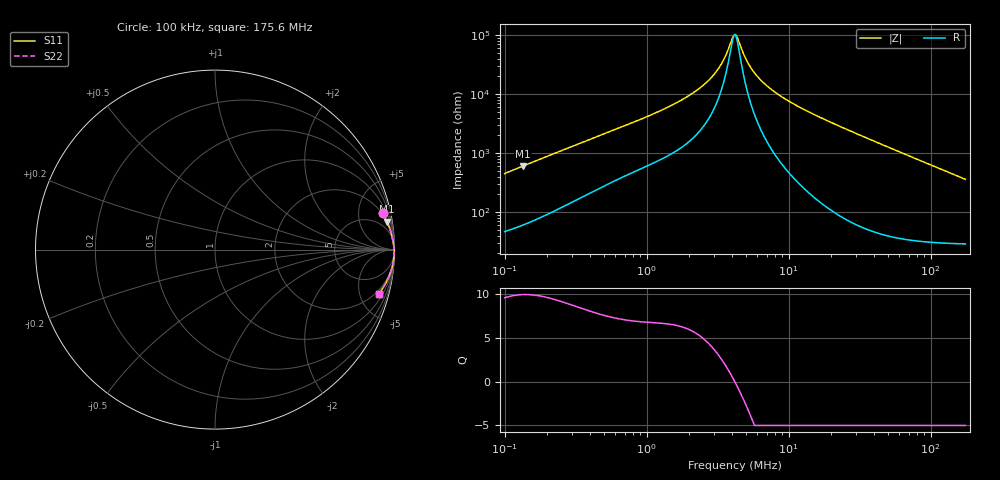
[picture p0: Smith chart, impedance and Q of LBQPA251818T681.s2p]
! LBQPA251818T681  S-PARAMETER MODEL  ( General Type )
! Model Generated by TAIYO YUDEN Corporation (http://www.ty-top.com)
! Version 1.0
! TAIYO YUDEN Control No. 191025NI43SB-FBB
! Copyright(c) 2019 TAIYO YUDEN CO.,LTD. All Rights Reserved.
! Product Description (link to TY-COMPAS)
! https://ds.yuden.co.jp/TYCOMPAS/or/detail?pn=LBQPA251818T681K&u=M
! Products Name : Inductors
! Characteristics :
!  Inductance : 680 uH , SRF(min) : 3.0 MHz , DC Resistance(max) : 36.4 Ohm
!  Rated Current : Saturation :65 mA , Temp Rise : 45 mA (20 degC)
!  Case Size : 2.5 x 1.8 / 0.098 x 0.071 [mm/inch] , Thickness : 1.8 / 0.071 [mm/inch]
!  (Conditions: Temperature = 25 degC , DC Bias Current/Voltage = 0A / 0V)
! External Node Assignments :
!  1  o---GGG---o  2
! GND o---------o GND
! Frequency Range : 0.1MHz  -  175.64884MHz  [ 402 STEP ]
# MHz S RI R 50
! Freq[MHz].  S11 Real  S11 Imag  S21 Real  S21 Imag  S12 Real  S12 Imag  S22 Real  S22 Imag
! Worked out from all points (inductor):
!   401 points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, 100 kHz to 175.6 MHz, reference 50 ohm
!   read as one part in series: L = 710 uH near 103.8 kHz
!   highest Q = 9.95 at 134.8 kHz (marker M1), where L = 710 uH
!   self-resonance near 4.113 MHz
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0.1  0.9342 0.2012  0.0658 -0.2012  0.0658 -0.2012  0.9342 0.2012
0.13483  0.9586 0.1552  0.0414 -0.1552  0.0414 -0.1552  0.9586 0.1552
0.349525  0.988 0.0646  0.012 -0.0646  0.012 -0.0646  0.988 0.0646
1.221676  0.9967 0.0193  0.00326 -0.0193  0.00326 -0.0193  0.9967 0.0193
1.948707  0.9981 0.0107  0.0019 -0.0107  0.0019 -0.0107  0.9981 0.0107
2.676973  0.9986 0.00596  0.00136 -0.00596  0.00136 -0.00596  0.9986 0.00596
2.994426  0.9988 0.00442  0.00123 -0.00442  0.00123 -0.00442  0.9988 0.00442
3.287545  0.9989 0.00316  0.00114 -0.00316  0.00114 -0.00316  0.9989 0.00316
3.609356  0.9989 0.00192  0.00106 -0.00192  0.00106 -0.00192  0.9989 0.00192
4.037378  0.999 0.000448  0.000993 -0.000448  0.000993 -0.000448  0.999 0.000448
4.191048  0.999 -4.2e-05  0.000974 4.2e-05  0.000974 4.2e-05  0.999 -4.2e-05
4.270063  0.999 -0.000287  0.000965 0.000287  0.000965 0.000287  0.999 -0.000287
4.432589  0.9991 -0.000778  0.000948 0.000778  0.000948 0.000778  0.9991 -0.000778
4.866487  0.9991 -0.00202  0.000913 0.00202  0.000913 0.00202  0.9991 -0.00202
5.243992  0.9991 -0.00302  0.000893 0.00302  0.000893 0.00302  0.9991 -0.00302
5.757316  0.9991 -0.0043  0.000877 0.0043  0.000877 0.0043  0.9991 -0.0043
6.440058  0.9991 -0.00589  0.00087 0.00589  0.00087 0.00589  0.9991 -0.00589
9.01361  0.9991 -0.0112  0.00093 0.0112  0.00093 0.0112  0.9991 -0.0112
14.64875  0.9987 -0.0213  0.00131 0.0213  0.00131 0.0213  0.9987 -0.0213
51.20104  0.9911 -0.0797  0.00895 0.0797  0.00895 0.0797  0.9911 -0.0797
104.1166  0.966 -0.1577  0.034 0.1577  0.034 0.1577  0.966 -0.1577
175.6488  0.9113 -0.2468  0.0887 0.2468  0.0887 0.2468  0.9113 -0.2468
